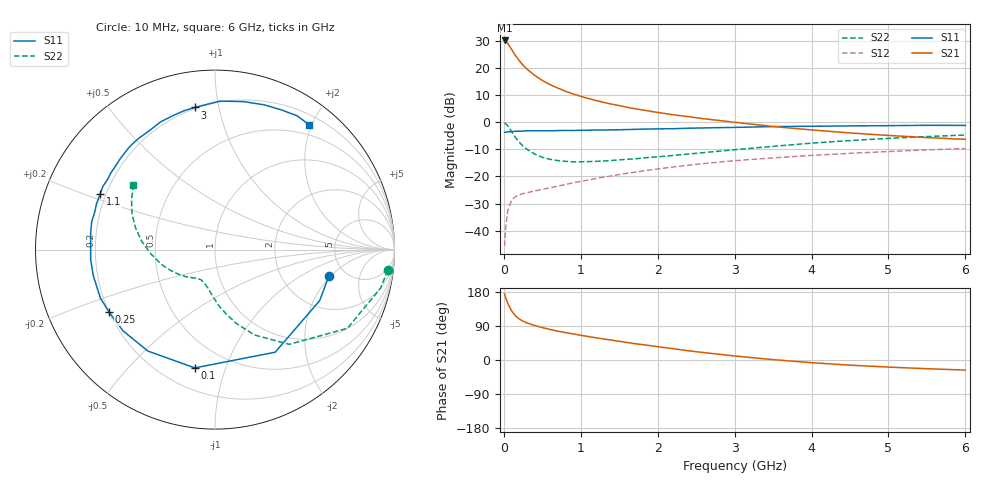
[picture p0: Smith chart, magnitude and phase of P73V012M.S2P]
! SIEMENS Small Signal Semiconductors
! BFP196
! Si NPN RF Bipolar Junction Transistor in SOT143
! VCE = 3 V  IC = 12 mA
! Common Emitter S-Parameters:  May  1996
# GHz  S  MA  R  50
!  f  S11  S21  S12  S22
! GHz  MAG  ANG  MAG  ANG  MAG  ANG  MAG  ANG
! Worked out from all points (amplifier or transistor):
!   36 points, 10 MHz to 6 GHz, reference 50 ohm
!   highest |S21| = 30.1 dB at 10 MHz (marker M1)
!   |S21| within 3 dB of that: start of sweep to 94.24 MHz
!   unconditionally stable (mu >= 1): 828.9 MHz to 3.316 GHz
!   at 250 MHz: K = 0.45, MSG = 23.6 dB, |S12| = -26.3 dB
!   at 1.4 GHz: K = 1.14, MAG = 10.9 dB, |S12| = -19.8 dB
!   at 6 GHz: K = 0.98, MSG = 1.7 dB, |S12| = -9.7 dB
!   S11 on the Smith chart (normalised r, x): 10 MHz: 3.68, -1.91; 100 MHz: 0.33, -0.79; 250 MHz: 0.20, -0.26; 1.1 GHz: 0.18, +0.22; 3 GHz: 0.19, +0.85; 6 GHz: 0.34, +1.97
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0.01  0.6511 -13.3  31.93 174.3  0.0052 86.0  0.9699 -6.8
0.02  0.6488 -26.0  31.12 166.9  0.0101 76.8  0.9473 -13.1
0.05  0.6628 -59.6  28.22 150.2  0.0231 64.9  0.8583 -30.7
0.1  0.6686 -99.7  21.96 129.8  0.0362 48.9  0.6709 -51.9
0.15  0.6778 -123.5  16.94 116.6  0.0426 41.1  0.5239 -65.2
0.2  0.6836 -138.5  13.6 108.3  0.0459 37.2  0.4281 -73.9
0.25  0.685 -149.4  11.18 102.2  0.0483 35.2  0.3606 -80.5
0.3  0.6933 -157.0  9.516 97.8  0.0502 34.6  0.3172 -85.6
0.4  0.6936 -168.1  7.294 91.0  0.0539 35.7  0.2583 -93.2
0.5  0.6949 -175.5  5.852 85.6  0.0579 37.3  0.2252 -98.7
0.6  0.6937 177.6  4.919 80.6  0.0618 39.2  0.2069 -103.6
0.8  0.7043 167.3  3.714 72.4  0.071 42.1  0.1897 -111.6
0.9  0.7019 162.7  3.307 68.8  0.0763 43.4  0.1858 -114.3
1.1  0.7103 154.2  2.722 61.8  0.086 45.0  0.1879 -119.4
1.3  0.7149 146.9  2.307 55.3  0.0972 45.8  0.1923 -124.6
1.6  0.7308 136.7  1.878 46.3  0.1142 46.1  0.2067 -132.0
2.2  0.757 118.8  1.367 29.8  0.1495 42.9  0.2437 -145.4
3  0.8002 98.2  0.994 10.6  0.1952 35.3  0.3107 -164.9
3.5  0.8281 88.0  0.832 1.0  0.2199 29.6  0.3585 -176.3
4.5  0.8522 71.1  0.632 -13.6  0.2669 18.7  0.4583 164.8
5.5  0.8747 58.5  0.519 -23.0  0.3082 7.4  0.5426 149.0
6  0.8708 52.8  0.483 -26.6  0.3267 1.5  0.5789 141.7
